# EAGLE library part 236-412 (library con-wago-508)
Terminal Strips 2.5 mm2/AWG 12, Series 236, Pin Spacings 5/5.08 mm Source: Data sheet
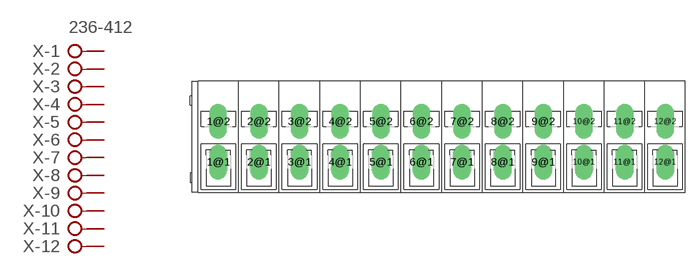
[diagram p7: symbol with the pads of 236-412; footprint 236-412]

Designator prefix X; gates -1=KL+V2 -2=KL+2 -3=KL+2 -4=KL+2 -5=KL+2 -6=KL+2 -7=KL+2 -8=KL+2 -9=KL+2 -10=KL+2 -11=KL+2 -12=KL+2

## 236-412 (MF: Wago Corporation; MPN: 0236-0412; OC_FARNELL: 1283531; OC_NEWARK: 79K2064)  [236-412]
1@1  -1:KL1  pas
1@2  -1:KL2  pas
2@1  -2:KL1  pas
2@2  -2:KL2  pas
3@1  -3:KL1  pas
3@2  -3:KL2  pas
4@1  -4:KL1  pas
4@2  -4:KL2  pas
5@1  -5:KL1  pas
5@2  -5:KL2  pas
6@1  -6:KL1  pas
6@2  -6:KL2  pas
7@1  -7:KL1  pas
7@2  -7:KL2  pas
8@1  -8:KL1  pas
8@2  -8:KL2  pas
9@1  -9:KL1  pas
9@2  -9:KL2  pas
10@1  -10:KL1  pas
10@2  -10:KL2  pas
11@1  -11:KL1  pas
11@2  -11:KL2  pas
12@1  -12:KL1  pas
12@2  -12:KL2  pas

## Footprint 236-412 (pad centres in mm)
Terminal Strips 2.5 mm2/AWG 12, Series 236, Pin Spacings 5/5.08 mm Source: Data sheet
drill 1.118 pad 2.184 long: 1@1 0,-2.54; 1@2 0,2.54; 2@1 5.08,-2.54; 2@2 5.08,2.54; 3@1 10.16,-2.54; 3@2 10.16,2.54; 4@1 15.24,-2.54; 4@2 15.24,2.54; 5@1 20.32,-2.54; 5@2 20.32,2.54; 6@1 25.4,-2.54; 6@2 25.4,2.54; 7@1 30.48,-2.54; 7@2 30.48,2.54; 8@1 35.56,-2.54; 8@2 35.56,2.54; 9@1 40.64,-2.54; 9@2 40.64,2.54; 10@1 45.72,-2.54; 10@2 45.72,2.54; 11@1 50.8,-2.54; 11@2 50.8,2.54; 12@1 55.88,-2.54; 12@2 55.88,2.54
